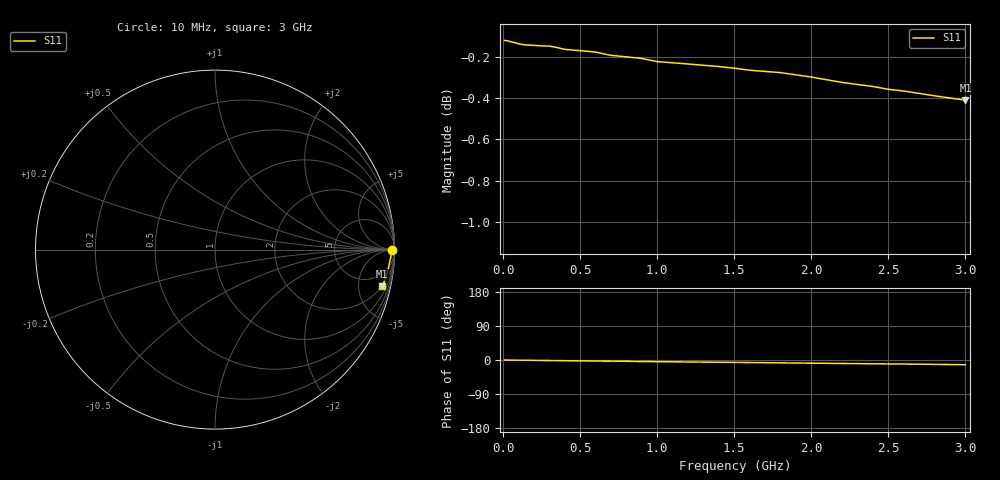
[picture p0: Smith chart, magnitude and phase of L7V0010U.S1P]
! SIEMENS Small Signal Semiconductors
! BAR14-1
! Si PIN Diode in SOT23
! IF = 0.01 mA
! S-Parameters:  July  1992
# GHz  S  MA  R  50
!  f  S11
! GHz  MAG  ANG
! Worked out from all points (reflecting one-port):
!   31 points, 10 MHz to 3 GHz, reference 50 ohm
!   lowest |S11| = -0.4 dB at 3 GHz (marker M1), VSWR 42.48, Z = 96.4 - j439 ohm
!   phase of S11 starts at -0 deg and turns -12 deg over the sweep
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0.01  0.9864 -0.1
0.03  0.9862 -0.2
0.05  0.9857 -0.3
0.06  0.9855 -0.4
0.08  0.9852 -0.5
0.1  0.9845 -0.5
0.15  0.9839 -0.7
0.2  0.9837 -1.0
0.3  0.9833 -1.4
0.4  0.9815 -1.8
0.5  0.9808 -2.2
0.6  0.98 -2.7
0.7  0.9782 -3.1
0.8  0.9774 -3.5
0.9  0.9765 -4.0
1  0.9748 -4.4
1.2  0.9735 -5.2
1.4  0.9721 -5.9
1.5  0.9712 -6.3
1.6  0.9701 -6.7
1.8  0.9688 -7.5
2  0.9664 -8.3
2.2  0.9635 -9.2
2.4  0.9613 -10.0
2.5  0.9598 -10.4
2.6  0.9589 -10.7
2.8  0.9563 -11.6
3  0.954 -12.4
